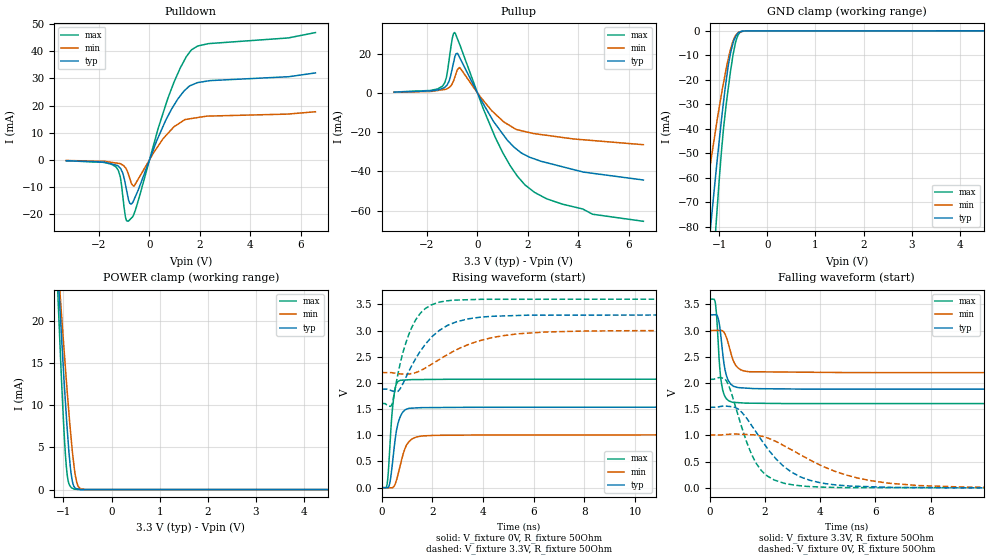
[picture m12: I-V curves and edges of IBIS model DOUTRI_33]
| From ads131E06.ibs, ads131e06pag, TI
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|   DOUTRI 3.3V Model
[Model]   DOUTRI_33
Model_type   I/O
|for all products
|Signals   DOUT, _DRDY
Vinl = 0.66
Vinh = 2.64
Vmeas = 1.65
Vref = 1.65
Cref = 2pF
Rref = 50
|   typ   min   max
|   (nom PVT)   (Fast PVT)   (slow PVT)
|C_comp from frequency sweep method (F=64MHz)
|   (Hight Z)
|C_comp   2.9770670e-12   2.2047960e-12   3.6911500e-12
|   (ON state)
|C_comp   5.1899950e-12   4.2044280e-12   5.9076290e-12
|   (OFF state)
|C_comp   6.1203700e-12   5.0777520e-12   7.3057800e-12
|C_comp from LC tank measurement(L=1nH)
|   (HIGH Z)
|C_comp   2.366E-12   1.803E-12   2.938E-12
|   (ON state)
C_comp   2.421E-12   1.888E-12   2.993E-12
|   (OFF state)
|C_comp   2.571E-12   1.871E-12   3.048E-12
| Where   nom PVT is  Nominal Process, 3.3V, 27C
|   Fast PVT is Strong Process, 3.6V, -40C
|   Slow PVT is Weak Process, 3V, 85C
[Voltage Range]   3.3   3   3.6
[Temperature Range]   27   85   -40
[Pullup Reference]   3.3   3   3.6
[Pulldown Reference]   0   0   0
[Power Clamp Reference]   3.3   3   3.6
[GND Clamp Reference]   0   0   0
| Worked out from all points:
|   slope of the pulldown table from 0 to 0.495 V, typ, clamps not added: 43.2 ohm
|   slope of the pullup table from 0 to 0.495 V, typ, clamps not added: 43.3 ohm
|   GND clamp passes 1 mA (typ) near -0.61 V on its own axis
|   POWER clamp passes 1 mA (typ) near -0.81 V on its own axis
|   falling waveform, V_fixture 3.3V, R_fixture 50Ohm: 20-80 % time 217ps typ, 293ps min, 163ps max; typ from 3.3 V to 1.88 V
|   rising waveform, V_fixture 0V, R_fixture 50Ohm: 20-80 % time 259ps typ, 357ps min, 182ps max; typ from 0 V to 1.54 V
|   rising waveform, V_fixture 3.3V, R_fixture 50Ohm: 20-80 % time 1.31ns typ, 2.17ns min, 763ps max; typ from 1.88 V to 3.3 V
|   falling waveform, V_fixture 0V, R_fixture 50Ohm: 20-80 % time 1.48ns typ, 2.58ns min, 882ps max; typ from 1.54 V to 0 V
[Pulldown]
|   Voltage   I(typ)   I(min)   I(max)
-3.3V     -285.2uA   -205.1uA   -305.9uA
-1.329V   -1.913mA   -1.131mA   -2.569mA
-1.166V   -2.978mA   -1.356mA   -5.896mA
-1.06V    -4.82mA    -1.891mA   -13.1mA
-952.1mV  -9.069mA   -2.877mA   -20.96mA
-845.4mV  -13.99mA   -4.934mA   -22.59mA
-726.6mV  -16.25mA   -8.344mA   -21.5mA
-602.2mV  -14.42mA   -9.513mA   -19.6mA
714.6mV   15.8mA     9.567mA    22.21mA
1.217V    23.5mA     13.68mA    33.7mA
1.659V    27.48mA    15.22mA    40.41mA
6.59V     32.02mA    17.73mA    46.86mA
[GND Clamp]
|   Voltage   I(typ)   I(min)   I(max)
-3.3V     -576.9mA   -412mA     -794.6mA
-1.359V   -118.2mA   -79.04mA   -168.2mA
-1.167V   -77.39mA   -52.12mA   -108.8mA
-1.06V    -56.05mA   -38.45mA   -77.2mA
-959mV    -37.13mA   -26.45mA   -50.3mA
-851.6mV  -19.7mA    -15.07mA   -29.37mA
-760.2mV  -8.518mA   -7.228mA   -15.77mA
-713.5mV  -5.047mA   -4.21mA    -9.784mA
-655.7mV  -2.214mA   -1.78mA    -4.311mA
-595.7mV  -679.8uA   -490.3uA   -1.367mA
-452.4mV  -21.29uA   -45.3uA    -19.88uA
6.59V     0A         0A         0A
[Pullup]
|   Voltage   I(typ)   I(min)   I(max)
-3.3V     365.8uA    284.3uA    421.3uA
-1.385V   2.267mA    1.566mA    3.423mA
-1.234V   3.548mA    1.87mA     7.54mA
-1.123V   5.879mA    2.67mA     16.59mA
-989.8mV  12.76mA    4.814mA    28.02mA
-901.9mV  17.87mA    7.684mA    30.71mA
-802.8mV  20.16mA    11.46mA    27.96mA
-682mV    17.5mA     12.65mA    24.04mA
714.6mV   -15.85mA   -10.81mA   -22.78mA
1.865V    -31.42mA   -19.63mA   -46.53mA
4.576V    -40.98mA   -24.29mA   -61.84mA
6.59V     -44.4mA    -26.41mA   -65.43mA
[POWER Clamp]
|   Voltage   I(typ)   I(min)   I(max)
-3.3V     287.9mA    235.1mA    365.7mA
-1.115V   26mA       26.9mA     23.05mA
-1.053V   19.46mA    21.85mA    14.67mA
-989.8mV  13.19mA    16.82mA    7.1mA
-938.7mV  8.594mA    12.89mA    2.672mA
-901.9mV  5.67mA     10.22mA    1.049mA
-856.1mV  2.654mA    7.086mA    377.6uA
-817.4mV  1.071mA    4.694mA    174.3uA
-776.5mV  327.6uA    2.652mA    58.48uA
-689.5mV  63.34uA    354.3uA    5.291uA
-547mV    5.186uA    4.364uA    5.187uA
6.59V     0A         0A         0A
[Ramp]
R_load = 50
|   typ   min   max
dV/dt_r   0.922224/2.5849e-010   0.605473/3.54686e-010   1.24254/1.8143e-010
dV/dt_f   0.851352/2.16185e-010  0.481819/2.9162e-010   1.19615/1.62636e-010
[Falling Waveform]
V_fixture = 3.3V
V_fixture_min = 3V
V_fixture_max = 3.6V
R_fixture = 50Ohm
C_fixture = 0F
|   Time   V(typ)   V(min)   V(max)
0s        3.3V       3V         3.6V
210.3ps   3.302V     3.002V     3.51V
260.2ps   3.293V     3.002V     3.215V
365.5ps   3.068V     3.003V     2.292V
463.4ps   2.61V      2.996V     1.89V
601.5ps   2.153V     2.875V     1.702V
812.3ps   1.958V     2.493V     1.634V
1.014ns   1.914V     2.293V     1.626V
1.422ns   1.899V     2.215V     1.615V
15.89ns   1.881V     2.197V     1.606V
[Rising Waveform]
V_fixture = 0V
V_fixture_min = 0V
V_fixture_max = 0V
R_fixture = 50Ohm
C_fixture = 0F
|   Time   V(typ)   V(min)   V(max)
0s        4.946uV    1.872uV    2.191uV
211.5ps   -2.985mV   -2.475mV   65.26mV
331.5ps   121.4mV    -3.88mV    868.7mV
391.6ps   334.7mV    -4.584mV   1.33V
469.7ps   671.9mV    15.47mV    1.707V
570.2ps   1.055V     124.8mV    1.97V
723.8ps   1.344V     412.1mV    2.049V
1.078ns   1.515V     881.8mV    2.06V
1.593ns   1.527V     986.8mV    2.065V
15.89ns   1.537V     1.009V     2.071V
[Rising Waveform]
V_fixture = 3.3V
V_fixture_min = 3V
V_fixture_max = 3.6V
R_fixture = 50Ohm
C_fixture = 0F
|   Time   V(typ)   V(min)   V(max)
0s        1.881V     2.197V     1.606V
404.1ps   1.849V     2.195V     1.589V
638.3ps   1.838V     2.176V     2.165V
835ps     1.984V     2.168V     2.577V
1.308ns   2.437V     2.192V     3.177V
1.699ns   2.724V     2.277V     3.411V
2.225ns   2.983V     2.433V     3.536V
3.386ns   3.22V      2.726V     3.589V
5.445ns   3.289V     2.94V      3.597V
15.89ns   3.3V       3V         3.6V
[Falling Waveform]
|Gnd
V_fixture = 0V
V_fixture_min = 0V
V_fixture_max = 0V
R_fixture = 50Ohm
C_fixture = 0F
|   Time   V(typ)   V(min)   V(max)
0s        1.537V     1.009V     2.071V
595.4ps   1.56V      1.017V     2.05V
1.05ns    1.496V     1.024V     1.349V
1.345ns   1.325V     1.017V     868.5mV
1.656ns   1.084V     1.007V     496.5mV
2.072ns   768.1mV    956.4mV    232.5mV
2.695ns   404.6mV    802.8mV    87.87mV
4.025ns   95.19mV    428.8mV    14.92mV
6.466ns   10.89mV    90.67mV    4.541mV
15.89ns   4.946uV    1.872uV    2.191uV
